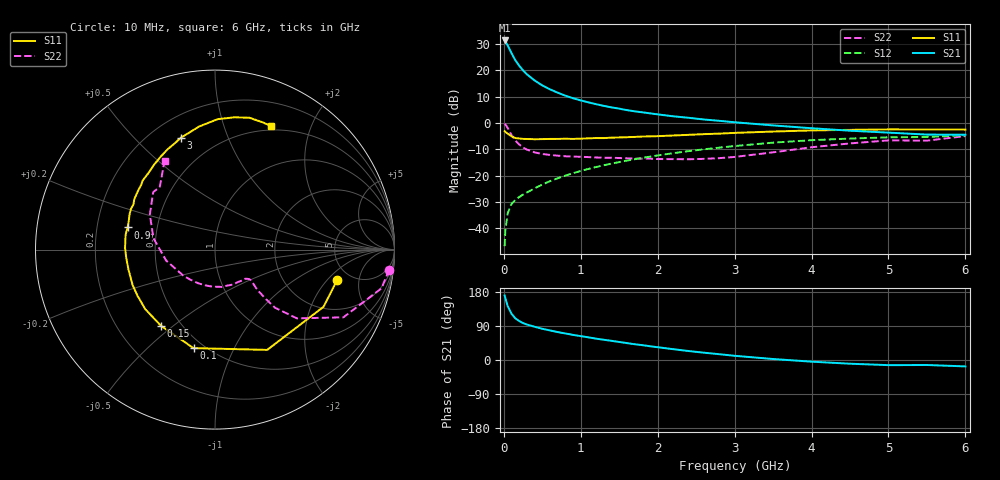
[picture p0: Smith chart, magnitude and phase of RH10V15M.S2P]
! SIEMENS Small Signal Semiconductors
! BFR106
! Si NPN RF Bipolar Junction Transistor in SOT23
! VCE = 10 V  IC = 15 mA
! Common Emitter S-Parameters:  August  1996
# GHz  S  MA  R  50
!  f  S11  S21  S12  S22
! GHz  MAG  ANG  MAG  ANG  MAG  ANG  MAG  ANG
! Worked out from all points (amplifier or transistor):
!   36 points, 10 MHz to 6 GHz, reference 50 ohm
!   highest |S21| = 31.4 dB at 10 MHz (marker M1)
!   |S21| within 3 dB of that: start of sweep to 68.67 MHz
!   unconditionally stable (mu >= 1): 431.5 MHz to 2.057 GHz
!   at 250 MHz: K = 0.80, MSG = 23.6 dB, |S12| = -27.1 dB
!   at 1.4 GHz: K = 1.07, MAG = 9.0 dB, |S12| = -15.4 dB
!   at 6 GHz: K = 0.99, MSG = 0.1 dB, |S12| = -4.6 dB
!   S11 on the Smith chart (normalised r, x): 10 MHz: 3.90, -2.59; 100 MHz: 0.44, -0.71; 150 MHz: 0.39, -0.46; 900 MHz: 0.34, +0.11; 3 GHz: 0.32, +0.69; 6 GHz: 0.46, +1.46
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0.01  0.7019 -13.9  37.2 170.4  0.0046 84.5  0.9768 -6.6
0.02  0.6835 -27.8  35.82 162.9  0.0093 78.0  0.9524 -13.1
0.05  0.63 -62.5  29.9 142.2  0.0194 63.0  0.8089 -27.8
0.1  0.5617 -102.3  21.29 121.9  0.0292 54.8  0.596 -40.0
0.15  0.5207 -125.1  15.62 109.8  0.0347 51.2  0.4652 -44.1
0.2  0.5108 -139.6  12.32 102.8  0.0395 52.4  0.3939 -44.2
0.25  0.5025 -149.3  10.04 97.3  0.044 53.6  0.3427 -43.7
0.3  0.4998 -156.7  8.467 93.6  0.0481 56.0  0.3142 -43.1
0.4  0.4948 -167.2  6.464 87.7  0.0579 59.2  0.2782 -41.3
0.5  0.4967 -174.7  5.208 82.4  0.0679 61.6  0.2592 -40.4
0.6  0.5011 179.1  4.382 78.0  0.0791 63.2  0.2491 -41.1
0.7  0.5022 174.1  3.79 73.7  0.0896 64.5  0.2412 -42.4
0.9  0.5022 165.8  2.972 66.3  0.1122 65.0  0.2315 -45.1
1.1  0.5148 157.7  2.48 59.7  0.1351 65.0  0.2262 -50.7
1.3  0.5196 151.0  2.126 53.4  0.1585 64.0  0.2205 -56.3
1.6  0.5407 142.1  1.766 44.6  0.1942 61.9  0.2148 -67.1
2.2  0.5821 125.7  1.349 28.6  0.2685 55.8  0.2073 -93.7
3  0.6523 106.8  1.039 11.1  0.3673 45.2  0.2279 -139.8
3.5  0.6925 97.1  0.906 2.6  0.426 37.6  0.2788 -167.3
4.5  0.7451 81.6  0.718 -9.8  0.5095 21.1  0.4121 151.8
5.5  0.7575 69.3  0.606 -13.2  0.5464 9.5  0.4656 131.3
6  0.7551 65.4  0.602 -16.9  0.5876 1.6  0.5677 119.7
